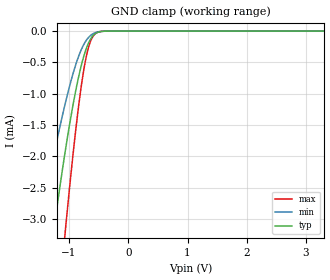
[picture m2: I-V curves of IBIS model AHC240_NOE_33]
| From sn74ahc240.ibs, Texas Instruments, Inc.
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[Model]   AHC240_NOE_33
Model_type  Input
Vinl=0.9
Vinh=2.1
| variable   typ   min   max
C_comp   0.60pF   0.52pF   0.68pF
[Temperature Range]   40   100   -40
| Ambient temperature   25   85   -40
[Voltage range]   3.3   3   3.6
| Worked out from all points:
|   GND clamp passes 1 mA (typ) near -0.90 V on its own axis
[GND Clamp]
| AHC240_NOE_33
|   Voltage   I(typ)   I(min)   I(max)
-5V       -42.63mA   -27.8mA    -54.13mA
-1.51V    -5.091mA   -3.226mA   -8.077mA
-1.255V   -3.17mA    -1.975mA   -5.195mA
-1.065V   -1.925mA   -1.161mA   -3.214mA
-895mV    -991.2uA   -561.3uA   -1.648mA
-835mV    -717.8uA   -394.5uA   -1.173mA
-770mV    -465.9uA   -248.7uA   -730.8uA
-720mV    -308.9uA   -163.3uA   -458.4uA
-670mV    -187.3uA   -100.6uA   -256.8uA
-560mV    -42.09uA   -26.19uA   -44.82uA
-405mV    -2.564uA   -1.802uA   -1.545uA
3.3V      3.885nA    645.3pA    18.64nA
